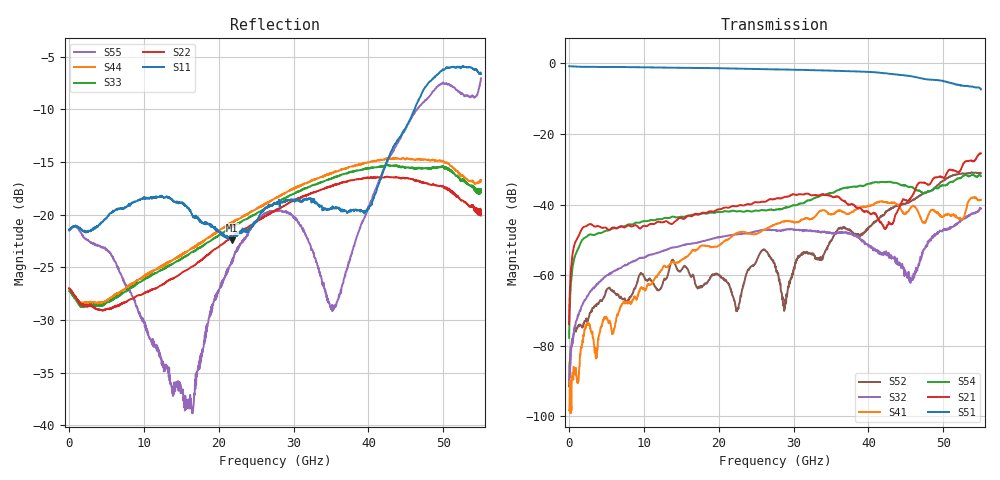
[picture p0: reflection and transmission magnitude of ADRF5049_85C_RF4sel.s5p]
! Device  : ADRF5049
! Description: Silicon SP4T Switch Non-Reflective
! Frequency:  9kHz -  45 GHz
! Ports:
!  RFC = Port 1
!  RF1 = Port 2
!  RF2 = Port 3
!	 RF3 = Port 4
!  RF4 = Port 5
! VSS  =  +3.30 Volts
! VDD  =  -3.30 Volts
! EN  =  0.00 Volts
! LS  =  0.00 Volts
! V1  =  3.30 Volts
! V2  =  3.30 Volts
! Data:  Data was collected using an calibrated 4 port network analyzer.
! Notes: Analog Devices supplies this data as a sample of measured data
!  for this product.  Your particular data for this product may vary.
!  Data was taken at 85 degrees C.
!  Analog Devices reserves the right to change this data at anytime.
# ghz S db R 50
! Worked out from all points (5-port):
!   1100 points, 50 MHz to 55 GHz, reference 50 ohm
!   strongest paths, dB at 50 MHz, 13.8 GHz, 27.55 GHz, 41.3 GHz, 55 GHz:
!     S51: -0.8, -1.3, -1.7, -2.6, -7.4
!     S21: -73.8, -45.5, -38.4, -44.1, -25.5
!     S54: -77.7, -43.4, -41.5, -33.7, -31.9
!     S41: -98.2, -56.3, -45.6, -39.4, -38.7
!     S32: -90.8, -52.1, -47.2, -53.8, -41.1
!     S52: -91.4, -55.7, -57.7, -44.0, -31.1
!   lowest |S11| = -22.4 dB at 21.75 GHz (marker M1), VSWR 1.16, Z = 55 + j6.16 ohm
!   |S11| at or under -10 dB: start of sweep to 46.16 GHz
